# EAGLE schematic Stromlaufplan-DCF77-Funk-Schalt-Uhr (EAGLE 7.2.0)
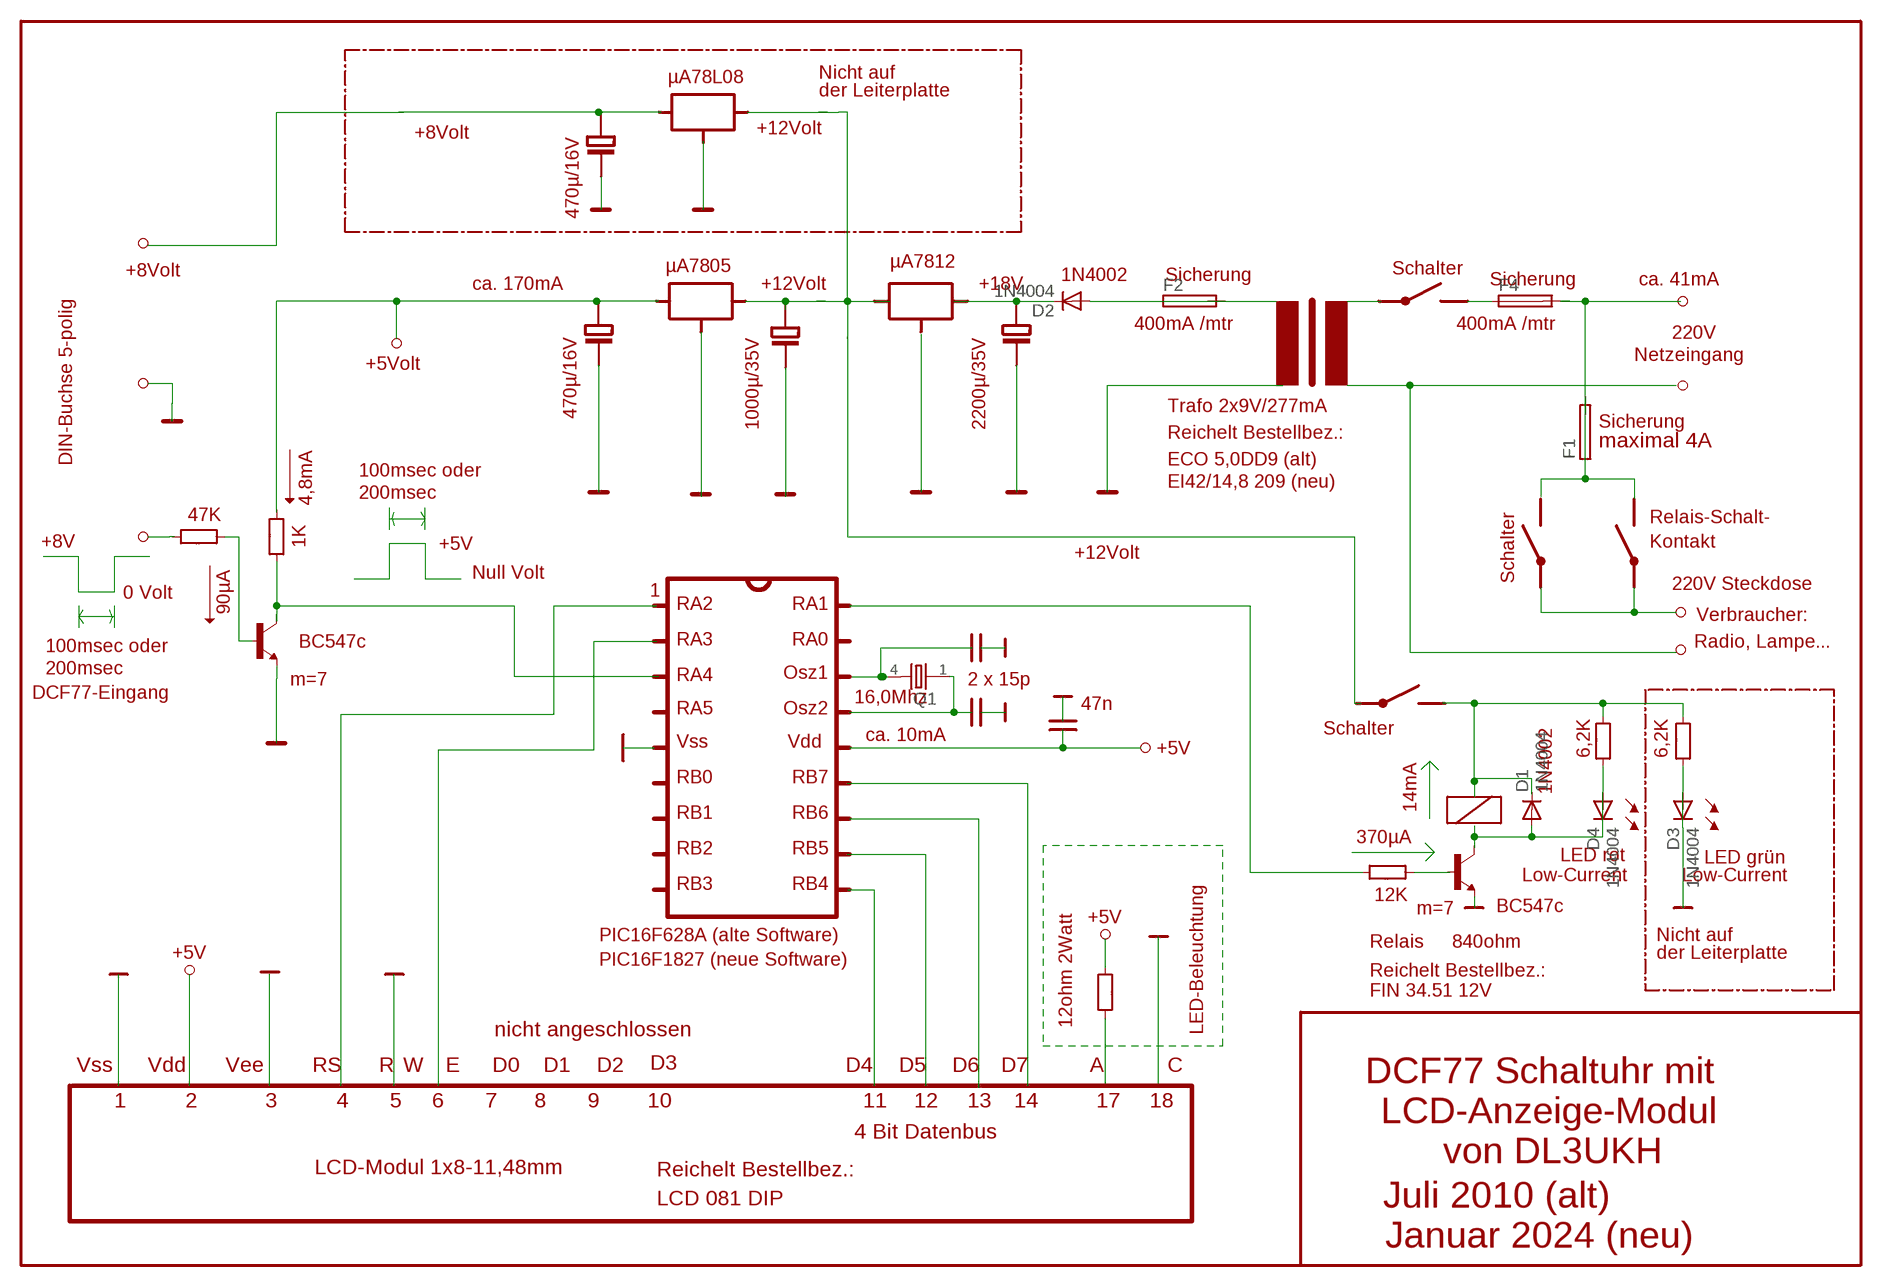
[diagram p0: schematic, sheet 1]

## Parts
D1  1N4004  [DO41-10]
D2  1N4004  [DO41-10]
D3  1N4004  [DO41-10]
D4  1N4004  [DO41-10]
F1  19559  [19559]
F2  19559  [19559]
F4  19559  [19559]
Q1  86SMX  [86SMX]

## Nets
N$6: D3.A D3.C
N$8: Q1.4
N$9: Q1.1
N$11: D2.C
N$15: D1.C
N$29: D1.A D4.A D4.C
N$36: D2.A F2.1 F2.2
N$48: F1.1 F1.2 F4.2
Unconnected: F4.1

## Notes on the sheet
- µA78L08 | Nicht auf
- der Leiterplatte
- +8Volt | +12Volt
- 470µ/16V
- Schalter
- µA7805 | µA7812
- +8Volt | 1N4002 | Sicherung
- ca. 170mA | +12Volt | +18V | Sicherung | ca. 41mA
- 400mA /mtr | 400mA /mtr
- 220V
- Netzeingang
- +5Volt
- Trafo 2x9V/277mA
- 470µ/16V
- 1000µ/35V | 2200µ/35V | Sicherung
- Reichelt Bestellbez.:
- maximal 4A
- DIN-Buchse 5-polig | ECO 5,0DD9 (alt)
- 100msec oder
- EI42/14,8 209 (neu)
- 200msec
- 4,8mA
- 47K | Relais-Schalt-
- +8V | 1K | +5V | Kontakt
- +12Volt
- Null Volt | Schalter
- 220V Steckdose
- 0 Volt | 1
- 90µA | RA2 | RA1
- Verbraucher:
- BC547c | RA3 | RA0 | Radio, Lampe...
- 100msec oder
- 200msec | Osz1
- m=7 | RA4 | 2 x 15p
- DCF77-Eingang | 16,0Mhz
- RA5 | Osz2 | 47n
- Schalter | 6,2K | 6,2K
- ca. 10mA
- Vss | Vdd
- +5V
- RB0 | RB7
- 1N4002
- 14mA
- RB1 | RB6
- 370µA | LED rot
- RB2 | RB5 | LED grün
- Low-Current | Low-Current
- RB3 | RB4
- 12K
- m=7 | BC547c
- PIC16F628A (alte Software) | +5V
- Nicht auf
- PIC16F1827 (neue Software) | Relais | 840ohm
- +5V | der Leiterplatte
- Reichelt Bestellbez.:
- FIN 34.51 12V
- 12ohm 2Watt
- nicht angeschlossen | LED-Beleuchtung
- Vss | Vdd | Vee | RS | R | W | E | D0 | D1 | D2 | D3 | D4 | D5 | D6 | D7 | A | C
- DCF77 Schaltuhr mit
- 1 | 2 | 3 | 4 | 5 | 6 | 7 | 8 | 9 | 10 | 11 | 12 | 13 | 14 | 17 | 18
- LCD-Anzeige-Modul
- 4 Bit Datenbus
- von DL3UKH
- LCD-Modul 1x8-11,48mm | Reichelt Bestellbez.:
- LCD 081 DIP | Juli 2010 (alt)
- Januar 2024 (neu)

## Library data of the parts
D1-D4 = diode:1N4004: DIODE
F1 F2 F4 = fuse:19559: FUSE HOLDER
Q1 = crystal:86SMX: CRYSTAL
